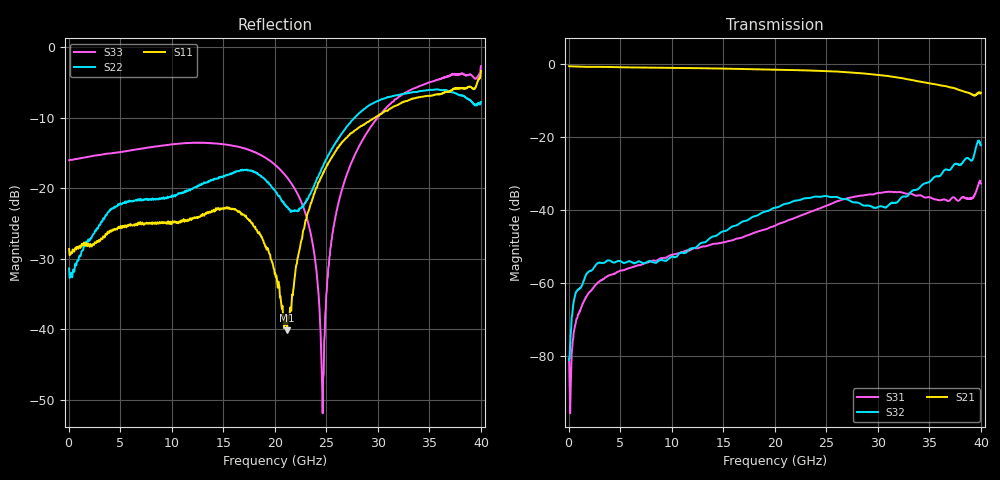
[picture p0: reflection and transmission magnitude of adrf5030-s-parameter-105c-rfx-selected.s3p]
! Device  : ADRF5030
! Description: Silicon SPDT Switch Non-Reflective
! Frequency:  100 MHz -  20 GHz
! Ports:
!  RFC = Port 1
!  RF1 = Port 2
!  RF2 = Port 3
! VSS  =  -3.30 Volts
! VDD  =  +3.30 Volts
! EN  =  0.00 Volts
! LS  =  0.00 Volts
! V1  =  +3.30 Volts
! Data:  Data was collected using an calibrated 4 port network analyzer.
! Notes: Analog Devices supplies this data as a sample of measured data
!  for this product.  Your particular data for this product may vary.
!  Data was taken at +105 degrees C.
!  Analog Devices reserves the right to change this data at anytime.
# HZ S DB R 50
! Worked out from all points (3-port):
!   800 points, 50 MHz to 40 GHz, reference 50 ohm
!   strongest paths, dB at 50 MHz, 10.05 GHz, 20.05 GHz, 30.05 GHz, 40 GHz:
!     S21: -0.5, -1.0, -1.5, -2.9, -7.8
!     S32: -81.1, -52.8, -39.3, -39.1, -22.2
!     S31: -80.8, -52.2, -44.2, -35.3, -32.7
!   lowest |S11| = -40.1 dB at 21.2 GHz (marker M1), VSWR 1.02, Z = 49.1 + j0.396 ohm
!   |S11| at or under -10 dB: start of sweep to 29.7 GHz
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5e7  -28.63 -2.6  -0.51 -0.2  -80.78 -34.7
     -0.51 -0.2  -31.37 -8.5  -81.06 10.6
     -80.78 -34.7  -81.06 10.6  -16.02 0.0
1.9e9  -27.87 -63.9  -0.69 -24.7  -62.96 82.7
       -0.69 -24.7  -27.27 -79.5  -56.98 45.8
       -62.96 82.7  -56.98 45.8  -15.54 -20.0
7.8e9  -24.98 148.6  -0.92 -101.1  -54.24 55.2
       -0.92 -101.1  -21.57 -146.4  -53.99 -4.9
       -54.24 55.2  -53.99 -4.9  -14.21 -82.0
1.395e10  -23.32 7.5  -1.12 179.4  -49.32 37.0
          -1.12 179.4  -18.78 -160.4  -47.27 -27.3
          -49.32 37.0  -47.27 -27.3  -13.62 -134.9
2.005e10  -32.07 -121.1  -1.48 97.2  -44.22 -0.1
          -1.48 97.2  -20.36 161.2  -39.32 -68.9
          -44.22 -0.1  -39.32 -68.9  -16.69 175.2
2.12e10  -40.13 155.8  -1.55 80.8  -42.90 -14.3
         -1.55 80.8  -22.61 170.5  -38.19 -78.5
         -42.90 -14.3  -38.19 -78.5  -18.48 166.0
2.465e10  -18.04 19.1  -1.81 30.4  -39.20 -67.0
          -1.81 30.4  -16.97 -145.4  -36.22 -116.2
          -39.20 -67.0  -36.22 -116.2  -51.92 -144.8
2.83e10  -11.25 -43.3  -2.44 -21.9  -36.02 -132.6
         -2.44 -21.9  -9.22 179.8  -38.24 176.4
         -36.02 -132.6  -38.24 176.4  -13.72 -90.5
3.655e10  -6.32 -152.3  -5.96 -128.9  -37.14 130.0
          -5.96 -128.9  -6.03 62.1  -28.87 -1.9
          -37.14 130.0  -28.87 -1.9  -4.21 154.2
4e10  -3.37 84.1  -7.80 130.9  -32.67 94.6
      -7.80 130.9  -7.76 -75.2  -22.23 -120.5
      -32.67 94.6  -22.23 -120.5  -2.69 14.2
